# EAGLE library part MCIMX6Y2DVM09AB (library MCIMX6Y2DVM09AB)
NXP - MCIMX6Y2DVM09AB - MPU, 32BIT, 900MHZ, 0 TO 95DEG C Source: Datasheet
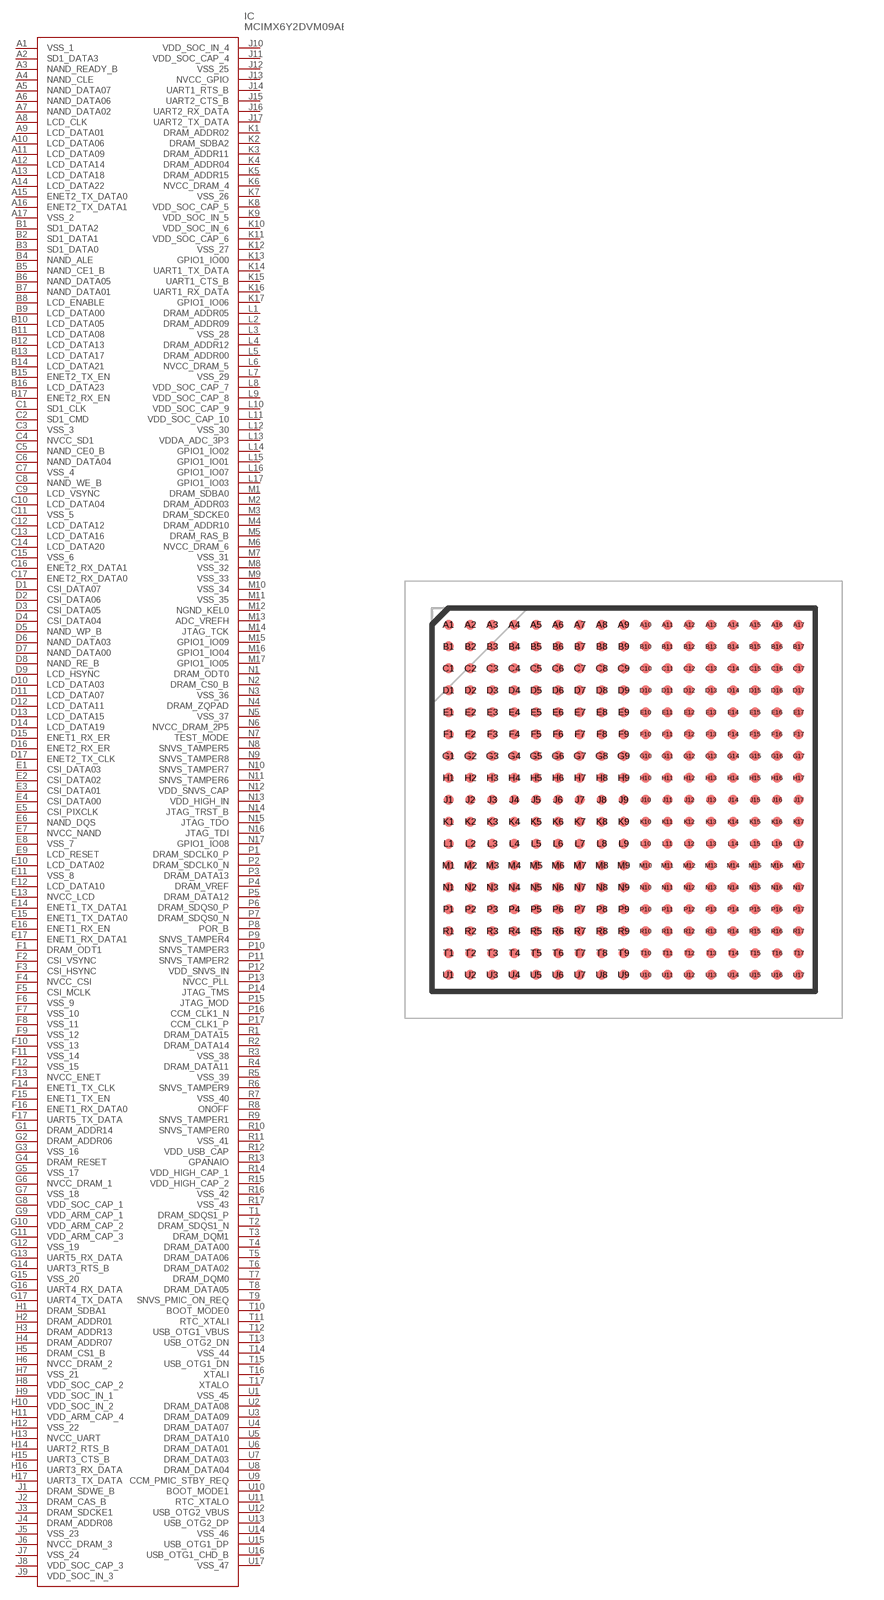
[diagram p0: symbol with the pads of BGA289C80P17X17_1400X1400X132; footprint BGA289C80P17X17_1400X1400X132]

Designator prefix IC

## MCIMX6Y2DVM09AB (Description: NXP - MCIMX6Y2DVM09AB - MPU, 32BIT, 900MHZ, 0 TO 95DEG C; Height: 1.32mm; Manufacturer_Name: NXP; Manufacturer_Part_Number: MCIMX6Y2DVM09AB; Mouser_Part_Number: 771-MCIMX6Y2DVM09AB; Mouser_Price-Stock: https://www.mouser.co.uk/ProductDetail/NXP-Semiconductors/MCIMX6Y2DVM09AB?qs=1mbolxNpo8dLZCzHiBeiHw%3D%3D)  [BGA289C80P17X17_1400X1400X132]
A1  VSS_1
A2  SD1_DATA3
A3  NAND_READY_B
A4  NAND_CLE
A5  NAND_DATA07
A6  NAND_DATA06
A7  NAND_DATA02
A8  LCD_CLK
A9  LCD_DATA01
A10  LCD_DATA06
A11  LCD_DATA09
A12  LCD_DATA14
A13  LCD_DATA18
A14  LCD_DATA22
A15  ENET2_TX_DATA0
A16  ENET2_TX_DATA1
A17  VSS_2
B1  SD1_DATA2
B2  SD1_DATA1
B3  SD1_DATA0
B4  NAND_ALE
B5  NAND_CE1_B
B6  NAND_DATA05
B7  NAND_DATA01
B8  LCD_ENABLE
B9  LCD_DATA00
B10  LCD_DATA05
B11  LCD_DATA08
B12  LCD_DATA13
B13  LCD_DATA17
B14  LCD_DATA21
B15  ENET2_TX_EN
B16  LCD_DATA23
B17  ENET2_RX_EN
C1  SD1_CLK
C2  SD1_CMD
C3  VSS_3
C4  NVCC_SD1
C5  NAND_CE0_B
C6  NAND_DATA04
C7  VSS_4
C8  NAND_WE_B
C9  LCD_VSYNC
C10  LCD_DATA04
C11  VSS_5
C12  LCD_DATA12
C13  LCD_DATA16
C14  LCD_DATA20
C15  VSS_6
C16  ENET2_RX_DATA1
C17  ENET2_RX_DATA0
D1  CSI_DATA07
D2  CSI_DATA06
D3  CSI_DATA05
D4  CSI_DATA04
D5  NAND_WP_B
D6  NAND_DATA03
D7  NAND_DATA00
D8  NAND_RE_B
D9  LCD_HSYNC
D10  LCD_DATA03
D11  LCD_DATA07
D12  LCD_DATA11
D13  LCD_DATA15
D14  LCD_DATA19
D15  ENET1_RX_ER
D16  ENET2_RX_ER
D17  ENET2_TX_CLK
E1  CSI_DATA03
E2  CSI_DATA02
E3  CSI_DATA01
E4  CSI_DATA00
E5  CSI_PIXCLK
E6  NAND_DQS
E7  NVCC_NAND
E8  VSS_7
E9  LCD_RESET
E10  LCD_DATA02
E11  VSS_8
E12  LCD_DATA10
E13  NVCC_LCD
E14  ENET1_TX_DATA1
E15  ENET1_TX_DATA0
E16  ENET1_RX_EN
E17  ENET1_RX_DATA1
F1  DRAM_ODT1
F2  CSI_VSYNC
F3  CSI_HSYNC
F4  NVCC_CSI
F5  CSI_MCLK
F6  VSS_9
F7  VSS_10
F8  VSS_11
F9  VSS_12
F10  VSS_13
F11  VSS_14
F12  VSS_15
F13  NVCC_ENET
F14  ENET1_TX_CLK
F15  ENET1_TX_EN
F16  ENET1_RX_DATA0
F17  UART5_TX_DATA
G1  DRAM_ADDR14
G2  DRAM_ADDR06
G3  VSS_16
G4  DRAM_RESET
G5  VSS_17
G6  NVCC_DRAM_1
G7  VSS_18
G8  VDD_SOC_CAP_1
G9  VDD_ARM_CAP_1
G10  VDD_ARM_CAP_2
G11  VDD_ARM_CAP_3
G12  VSS_19
G13  UART5_RX_DATA
G14  UART3_RTS_B
G15  VSS_20
G16  UART4_RX_DATA
G17  UART4_TX_DATA
H1  DRAM_SDBA1
H2  DRAM_ADDR01
H3  DRAM_ADDR13
H4  DRAM_ADDR07
H5  DRAM_CS1_B
H6  NVCC_DRAM_2
H7  VSS_21
H8  VDD_SOC_CAP_2
H9  VDD_SOC_IN_1
H10  VDD_SOC_IN_2
H11  VDD_ARM_CAP_4
H12  VSS_22
H13  NVCC_UART
H14  UART2_RTS_B
H15  UART3_CTS_B
H16  UART3_RX_DATA
H17  UART3_TX_DATA
J1  DRAM_SDWE_B
J2  DRAM_CAS_B
J3  DRAM_SDCKE1
J4  DRAM_ADDR08
J5  VSS_23
J6  NVCC_DRAM_3
J7  VSS_24
J8  VDD_SOC_CAP_3
J9  VDD_SOC_IN_3
J10  VDD_SOC_IN_4
J11  VDD_SOC_CAP_4
J12  VSS_25
J13  NVCC_GPIO
J14  UART1_RTS_B
J15  UART2_CTS_B
J16  UART2_RX_DATA
J17  UART2_TX_DATA
K1  DRAM_ADDR02
K2  DRAM_SDBA2
K3  DRAM_ADDR11
K4  DRAM_ADDR04
K5  DRAM_ADDR15
K6  NVCC_DRAM_4
K7  VSS_26
K8  VDD_SOC_CAP_5
K9  VDD_SOC_IN_5
K10  VDD_SOC_IN_6
K11  VDD_SOC_CAP_6
K12  VSS_27
K13  GPIO1_IO00
K14  UART1_TX_DATA
K15  UART1_CTS_B
K16  UART1_RX_DATA
K17  GPIO1_IO06
L1  DRAM_ADDR05
L2  DRAM_ADDR09
L3  VSS_28
L4  DRAM_ADDR12
L5  DRAM_ADDR00
L6  NVCC_DRAM_5
L7  VSS_29
L8  VDD_SOC_CAP_7
L9  VDD_SOC_CAP_8
L10  VDD_SOC_CAP_9
L11  VDD_SOC_CAP_10
L12  VSS_30
L13  VDDA_ADC_3P3
L14  GPIO1_IO02
L15  GPIO1_IO01
L16  GPIO1_IO07
L17  GPIO1_IO03
M1  DRAM_SDBA0
M2  DRAM_ADDR03
M3  DRAM_SDCKE0
M4  DRAM_ADDR10
M5  DRAM_RAS_B
M6  NVCC_DRAM_6
M7  VSS_31
M8  VSS_32
M9  VSS_33
M10  VSS_34
M11  VSS_35
M12  NGND_KEL0
M13  ADC_VREFH
M14  JTAG_TCK
M15  GPIO1_IO09
M16  GPIO1_IO04
M17  GPIO1_IO05
N1  DRAM_ODT0
N2  DRAM_CS0_B
N3  VSS_36
N4  DRAM_ZQPAD
N5  VSS_37
N6  NVCC_DRAM_2P5
N7  TEST_MODE
N8  SNVS_TAMPER5
N9  SNVS_TAMPER8
N10  SNVS_TAMPER7
N11  SNVS_TAMPER6
N12  VDD_SNVS_CAP
N13  VDD_HIGH_IN
N14  JTAG_TRST_B
N15  JTAG_TDO
N16  JTAG_TDI
N17  GPIO1_IO08
P1  DRAM_SDCLK0_P
P2  DRAM_SDCLK0_N
P3  DRAM_DATA13
P4  DRAM_VREF
P5  DRAM_DATA12
P6  DRAM_SDQS0_P
P7  DRAM_SDQS0_N
P8  POR_B
P9  SNVS_TAMPER4
P10  SNVS_TAMPER3
P11  SNVS_TAMPER2
P12  VDD_SNVS_IN
P13  NVCC_PLL
P14  JTAG_TMS
P15  JTAG_MOD
P16  CCM_CLK1_N
P17  CCM_CLK1_P
R1  DRAM_DATA15
R2  DRAM_DATA14
R3  VSS_38
R4  DRAM_DATA11
R5  VSS_39
R6  SNVS_TAMPER9
R7  VSS_40
R8  ONOFF
R9  SNVS_TAMPER1
R10  SNVS_TAMPER0
R11  VSS_41
R12  VDD_USB_CAP
R13  GPANAIO
R14  VDD_HIGH_CAP_1
R15  VDD_HIGH_CAP_2
R16  VSS_42
R17  VSS_43
T1  DRAM_SDQS1_P
T2  DRAM_SDQS1_N
T3  DRAM_DQM1
T4  DRAM_DATA00
T5  DRAM_DATA06
T6  DRAM_DATA02
T7  DRAM_DQM0
T8  DRAM_DATA05
T9  SNVS_PMIC_ON_REQ
T10  BOOT_MODE0
T11  RTC_XTALI
T12  USB_OTG1_VBUS
T13  USB_OTG2_DN
T14  VSS_44
T15  USB_OTG1_DN
T16  XTALI
T17  XTALO
U1  VSS_45
U2  DRAM_DATA08
U3  DRAM_DATA09
U4  DRAM_DATA07
U5  DRAM_DATA10
U6  DRAM_DATA01
U7  DRAM_DATA03
U8  DRAM_DATA04
U9  CCM_PMIC_STBY_REQ
U10  BOOT_MODE1
U11  RTC_XTALO
U12  USB_OTG2_VBUS
U13  USB_OTG2_DP
U14  VSS_46
U15  USB_OTG1_DP
U16  USB_OTG1_CHD_B
U17  VSS_47

## Footprint BGA289C80P17X17_1400X1400X132 (pad centres in mm)
MCIMX6Y2DVM09AB_11
smd 0.37 x 0.37: A1 -6.4,6.4; A2 -5.6,6.4; A3 -4.8,6.4; A4 -4,6.4; A5 -3.2,6.4; A6 -2.4,6.4; A7 -1.6,6.4; A8 -0.8,6.4; A9 0,6.4; A10 0.8,6.4; A11 1.6,6.4; A12 2.4,6.4; A13 3.2,6.4; A14 4,6.4; A15 4.8,6.4; A16 5.6,6.4; A17 6.4,6.4; B1 -6.4,5.6; B2 -5.6,5.6; B3 -4.8,5.6; B4 -4,5.6; B5 -3.2,5.6; B6 -2.4,5.6; B7 -1.6,5.6; B8 -0.8,5.6; B9 0,5.6; B10 0.8,5.6; B11 1.6,5.6; B12 2.4,5.6; B13 3.2,5.6; B14 4,5.6; B15 4.8,5.6; B16 5.6,5.6; B17 6.4,5.6; C1 -6.4,4.8; C2 -5.6,4.8; C3 -4.8,4.8; C4 -4,4.8; C5 -3.2,4.8; C6 -2.4,4.8; C7 -1.6,4.8; C8 -0.8,4.8; C9 0,4.8; C10 0.8,4.8; C11 1.6,4.8; C12 2.4,4.8; C13 3.2,4.8; C14 4,4.8; C15 4.8,4.8; C16 5.6,4.8; C17 6.4,4.8; D1 -6.4,4; D2 -5.6,4; D3 -4.8,4; D4 -4,4; D5 -3.2,4; D6 -2.4,4; D7 -1.6,4; D8 -0.8,4; D9 0,4; D10 0.8,4; D11 1.6,4; D12 2.4,4; D13 3.2,4; D14 4,4; D15 4.8,4; D16 5.6,4; D17 6.4,4; E1 -6.4,3.2; E2 -5.6,3.2; E3 -4.8,3.2; E4 -4,3.2; E5 -3.2,3.2; E6 -2.4,3.2; E7 -1.6,3.2; E8 -0.8,3.2; E9 0,3.2; E10 0.8,3.2; E11 1.6,3.2; E12 2.4,3.2; E13 3.2,3.2; E14 4,3.2; E15 4.8,3.2; E16 5.6,3.2; E17 6.4,3.2; F1 -6.4,2.4; F2 -5.6,2.4; F3 -4.8,2.4; F4 -4,2.4; F5 -3.2,2.4; F6 -2.4,2.4; F7 -1.6,2.4; F8 -0.8,2.4; F9 0,2.4; F10 0.8,2.4; F11 1.6,2.4; F12 2.4,2.4; F13 3.2,2.4; F14 4,2.4; F15 4.8,2.4; F16 5.6,2.4; F17 6.4,2.4; G1 -6.4,1.6; G2 -5.6,1.6; G3 -4.8,1.6; G4 -4,1.6; G5 -3.2,1.6; G6 -2.4,1.6; G7 -1.6,1.6; G8 -0.8,1.6; G9 0,1.6; G10 0.8,1.6; G11 1.6,1.6; G12 2.4,1.6; G13 3.2,1.6; G14 4,1.6; G15 4.8,1.6; G16 5.6,1.6; G17 6.4,1.6; H1 -6.4,0.8; H2 -5.6,0.8; H3 -4.8,0.8; H4 -4,0.8; H5 -3.2,0.8; H6 -2.4,0.8; H7 -1.6,0.8; H8 -0.8,0.8; H9 0,0.8; H10 0.8,0.8; H11 1.6,0.8; H12 2.4,0.8; H13 3.2,0.8; H14 4,0.8; H15 4.8,0.8; H16 5.6,0.8; H17 6.4,0.8; J1 -6.4,0; J2 -5.6,0; J3 -4.8,0; J4 -4,0; J5 -3.2,0; J6 -2.4,0; J7 -1.6,0; J8 -0.8,0; J9 0,0; J10 0.8,0; J11 1.6,0; J12 2.4,0; J13 3.2,0; J14 4,0; J15 4.8,0; J16 5.6,0; J17 6.4,0; K1 -6.4,-0.8; K2 -5.6,-0.8; K3 -4.8,-0.8; K4 -4,-0.8; K5 -3.2,-0.8; K6 -2.4,-0.8; K7 -1.6,-0.8; K8 -0.8,-0.8; K9 0,-0.8; K10 0.8,-0.8; K11 1.6,-0.8; K12 2.4,-0.8; K13 3.2,-0.8; K14 4,-0.8; K15 4.8,-0.8; K16 5.6,-0.8; K17 6.4,-0.8; L1 -6.4,-1.6; L2 -5.6,-1.6; L3 -4.8,-1.6; L4 -4,-1.6; L5 -3.2,-1.6; L6 -2.4,-1.6; L7 -1.6,-1.6; L8 -0.8,-1.6; L9 0,-1.6; L10 0.8,-1.6; L11 1.6,-1.6; L12 2.4,-1.6; L13 3.2,-1.6; L14 4,-1.6; L15 4.8,-1.6; L16 5.6,-1.6; L17 6.4,-1.6; M1 -6.4,-2.4; M2 -5.6,-2.4; M3 -4.8,-2.4; M4 -4,-2.4; M5 -3.2,-2.4; M6 -2.4,-2.4; M7 -1.6,-2.4; M8 -0.8,-2.4; M9 0,-2.4; M10 0.8,-2.4; M11 1.6,-2.4; M12 2.4,-2.4; M13 3.2,-2.4; M14 4,-2.4; M15 4.8,-2.4; M16 5.6,-2.4; M17 6.4,-2.4; N1 -6.4,-3.2; N2 -5.6,-3.2; N3 -4.8,-3.2; N4 -4,-3.2; N5 -3.2,-3.2; N6 -2.4,-3.2; N7 -1.6,-3.2; N8 -0.8,-3.2; N9 0,-3.2; N10 0.8,-3.2; N11 1.6,-3.2; N12 2.4,-3.2; N13 3.2,-3.2; N14 4,-3.2; N15 4.8,-3.2; N16 5.6,-3.2; N17 6.4,-3.2; P1 -6.4,-4; P2 -5.6,-4; P3 -4.8,-4; P4 -4,-4; P5 -3.2,-4; P6 -2.4,-4; P7 -1.6,-4; P8 -0.8,-4; P9 0,-4; P10 0.8,-4; P11 1.6,-4; P12 2.4,-4; P13 3.2,-4; P14 4,-4; P15 4.8,-4; P16 5.6,-4; P17 6.4,-4; R1 -6.4,-4.8; R2 -5.6,-4.8; R3 -4.8,-4.8; R4 -4,-4.8; R5 -3.2,-4.8; R6 -2.4,-4.8; R7 -1.6,-4.8; R8 -0.8,-4.8; R9 0,-4.8; R10 0.8,-4.8; R11 1.6,-4.8; R12 2.4,-4.8; R13 3.2,-4.8; R14 4,-4.8; R15 4.8,-4.8; R16 5.6,-4.8; R17 6.4,-4.8; T1 -6.4,-5.6; T2 -5.6,-5.6; T3 -4.8,-5.6; T4 -4,-5.6; T5 -3.2,-5.6; T6 -2.4,-5.6; T7 -1.6,-5.6; T8 -0.8,-5.6; T9 0,-5.6; T10 0.8,-5.6; T11 1.6,-5.6; T12 2.4,-5.6; T13 3.2,-5.6; T14 4,-5.6; T15 4.8,-5.6; T16 5.6,-5.6; T17 6.4,-5.6; U1 -6.4,-6.4; U2 -5.6,-6.4; U3 -4.8,-6.4; U4 -4,-6.4; U5 -3.2,-6.4; U6 -2.4,-6.4; U7 -1.6,-6.4; U8 -0.8,-6.4; U9 0,-6.4; U10 0.8,-6.4; U11 1.6,-6.4; U12 2.4,-6.4; U13 3.2,-6.4; U14 4,-6.4; U15 4.8,-6.4; U16 5.6,-6.4; U17 6.4,-6.4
